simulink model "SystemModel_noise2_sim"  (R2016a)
settings: Solver=FixedStepAuto  StartTime=0.0  StopTime=Endtime  FixedStep=0.05  RelTol=1e-3
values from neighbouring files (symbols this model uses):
  alpha_AD = (2^n_AD - 1)/(V_AD_max - V_AD_min)    (= 204.6)    [SystemModel_noise2.m]    (also in SystemModel_noise1.m)
  alpha_PG = 100/(2^n_PG-1)    (= 0.392156862745)    [SystemModel_noise2.m]    (also in SystemModel_noise1.m)
  alpha_S_i = 5/37.5    (= 0.133333333333)    [SystemModel_noise2.m]    (also in MotorDriver_m.m; SystemModel_noise1.m)
  alpha_S_N = 1.5/1000    (= 0.0015)    [SystemModel_noise2.m]    (also in SystemModel_noise1.m)
  D_R = 6.0e-5    (= 6e-05)    [SystemModel_noise2.m]    (also in SystemModel_noise1.m)
  J_I = 1.3e-3    (= 0.0013)    [SystemModel_noise2.m]    (also in DCMotorDisk.m; SystemModel_noise1.m)
  J_M = 0.11e-3    (= 0.00011)    [SystemModel_noise2.m]    (also in DCMotorDisk.m; SystemModel_noise1.m)
  K_E = 7.16e-2    (= 0.0716)    [SystemModel_noise2.m]    (also in SystemModel_noise1.m)
  K_tau = 7.2e-2    (= 0.072)    [SystemModel_noise2.m]    (also in DCMotorDisk.m; SystemModel_noise1.m)
  kc = 0.1    [SystemModel_noise2.m]    (also in SystemModel_noise1.m = 0.05)
  L_E = 0.2    [SystemModel_noise2.m]    (also in SystemModel_noise1.m)
  n_PG = 8    [SystemModel_noise2.m]    (also in SystemModel_noise1.m)
  R_E = 5.7    [SystemModel_noise2.m]    (also in SystemModel_noise1.m)
  SV = 1000    [SystemModel_noise2.m]    (also in SystemModel_noise1.m)
  T_D = 0.1    [SystemModel_noise2.m]    (also in SystemModel_noise1.m = 0.01)
  T_I = 1.5    [SystemModel_noise2.m]    (also in SystemModel_noise1.m = 1.2)
  Tc = 1/(2*pi*fc)    (= 0.159154943092)    [SystemModel_noise2.m]
  u_max = 100    [SystemModel_noise2.m]    (also in Controller.m; SystemModel_noise1.m)
  u_min = 0    [SystemModel_noise2.m]    (also in Controller.m; SystemModel_noise1.m)
  V_AD_max = 5    [SystemModel_noise2.m]    (also in SystemModel_noise1.m)
  V_AD_min = 0    [SystemModel_noise2.m]    (also in SystemModel_noise1.m)
  Vs = 24    [SystemModel_noise2.m]    (also in MotorDriver.m; MotorDriver_m.m; SystemModel_noise1.m)

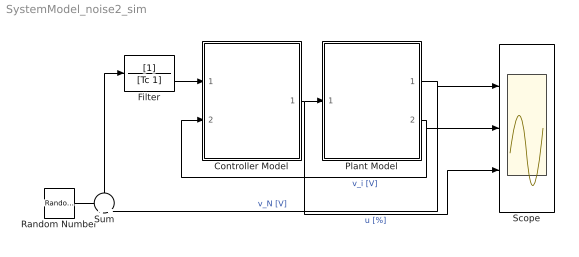
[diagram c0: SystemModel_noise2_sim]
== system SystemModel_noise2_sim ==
  Controller Model : Subsystem
  Filter : TransferFcn  Commented=through  Denominator=[Tc 1]
  Plant Model : Subsystem
  Random Number : RandomNumber  Variance=1e-2  SampleTime=0
  Scope : Scope  NumInputPorts=3
  Sum : Sum  Inputs=+|+
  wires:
  Controller Model/1(u_PG [%]) -> Scope/3, Plant Model/1(u_MD [%])  "u [%]"
  Plant Model/2(v_i [V]) -> Scope/2, Controller Model/2(v_i [V])  "v_i [V]"
  Plant Model/1(v_N [V]) -> Sum/2, Scope/1  "v_N [V]"
  Sum/1 -> Filter/1
  Random Number/1 -> Sum/1
  Filter/1 -> Controller Model/1(v_N [V])

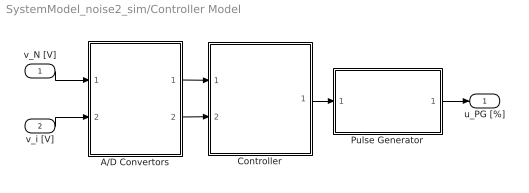
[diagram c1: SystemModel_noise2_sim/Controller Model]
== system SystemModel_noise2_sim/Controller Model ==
  v_N [V] : Inport
  v_i [V] : Inport  Port=2
  A/D Convertors : Subsystem
  Controller : Subsystem
  Pulse Generator : Subsystem
  u_PG [%] : Outport
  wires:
  v_i [V]/1 -> A/D Convertors/2(v_i [V])
  A/D Convertors/2(d_AD_i [-]) -> Controller/2(d_AD_i [-])
  Controller/1(d_PG [-]) -> Pulse Generator/1(d_PG [-])
  A/D Convertors/1(d_AD_N [-]) -> Controller/1(d_AD_N [-])
  Pulse Generator/1(u_PG [%]) -> u_PG [%]/1
  v_N [V]/1 -> A/D Convertors/1(v_N [V])

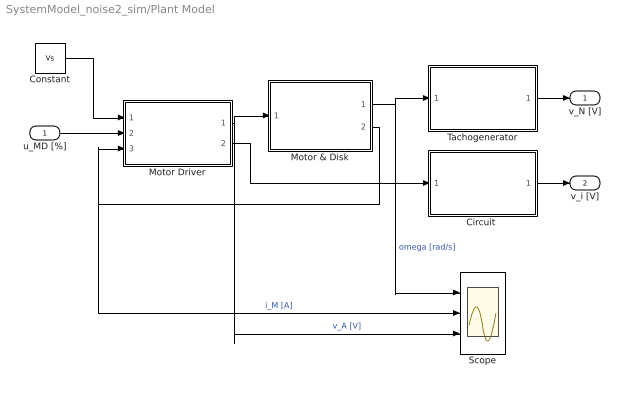
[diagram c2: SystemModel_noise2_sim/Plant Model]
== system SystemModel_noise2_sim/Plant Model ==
  u_MD [%] : Inport
  "Circuit " : Subsystem
  Constant : Constant  Value=Vs
  Motor & Disk : Subsystem
  Motor Driver : Subsystem
  Scope : Scope  NumInputPorts=3
  Tachogenerator : Subsystem
  v_N [V] : Outport
  v_i [V] : Outport  Port=2
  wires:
  Tachogenerator/1(v_N [V]) -> v_N [V]/1
  Motor Driver/1(v_A [V]) -> Scope/3, Motor & Disk/1(v_M [V])  "v_A [V]"
  Constant/1 -> Motor Driver/1(Vs [V])
  Motor & Disk/1(omega [rad/s]) -> Scope/1, Tachogenerator/1(omega [rad/s])  "omega [rad/s]"
  u_MD [%]/1 -> Motor Driver/2(u_MD [%])
  Motor & Disk/2(i_M [A]) -> Scope/2, Motor Driver/3(i_M [A])  "i_M [A]"
  Motor Driver/2(v_i [V]) -> "Circuit "/1(v_i [V])
  "Circuit "/1(v_i_st [V]) -> v_i [V]/1

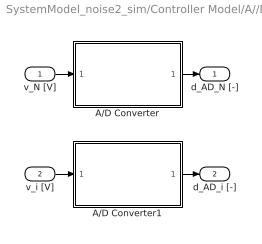
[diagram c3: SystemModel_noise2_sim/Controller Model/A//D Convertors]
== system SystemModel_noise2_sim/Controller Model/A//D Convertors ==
  v_N [V] : Inport
  v_i [V] : Inport  Port=2
  A/D Converter : Subsystem
  A/D Converter1 : Subsystem
  d_AD_N [-] : Outport
  d_AD_i [-] : Outport  Port=2
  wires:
  A/D Converter1/1(d_AD [-]) -> d_AD_i [-]/1
  v_N [V]/1 -> A/D Converter/1(v_AD [V])
  v_i [V]/1 -> A/D Converter1/1(v_AD [V])
  A/D Converter/1(d_AD [-]) -> d_AD_N [-]/1

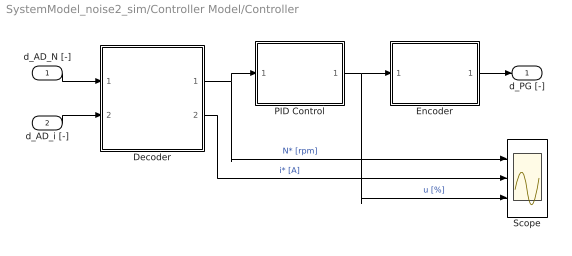
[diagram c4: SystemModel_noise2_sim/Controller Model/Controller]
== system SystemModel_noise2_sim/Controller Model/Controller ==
  d_AD_N [-] : Inport
  d_AD_i [-] : Inport  Port=2
  Decoder : Subsystem
  Encoder : Subsystem
  PID Control : Subsystem
  Scope : Scope  NumInputPorts=3
  d_PG [-] : Outport
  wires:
  d_AD_N [-]/1 -> Decoder/1(d_AD_N [-])
  Encoder/1(d_PG [-]) -> d_PG [-]/1
  Decoder/1(N* [rpm]) -> PID Control/1(N* [rpm]), Scope/1  "N* [rpm]"
  Decoder/2(i* [A]) -> Scope/2  "i* [A]"
  d_AD_i [-]/1 -> Decoder/2(d_AD_i [-])
  PID Control/1(u [%]) -> Scope/3, Encoder/1(u [%])  "u [%]"

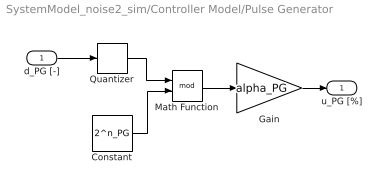
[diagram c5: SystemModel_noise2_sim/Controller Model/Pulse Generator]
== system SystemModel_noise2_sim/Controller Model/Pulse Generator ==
  d_PG [-] : Inport
  Constant : Constant  Value=2^n_PG
  Gain : Gain  Gain=alpha_PG
  Math Function : Math  Operator=mod
  Quantizer : Quantizer  QuantizationInterval=1
  u_PG [%] : Outport
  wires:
  d_PG [-]/1 -> Quantizer/1
  Quantizer/1 -> Math Function/1
  Gain/1 -> u_PG [%]/1
  Math Function/1 -> Gain/1
  Constant/1 -> Math Function/2

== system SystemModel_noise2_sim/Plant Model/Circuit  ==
  v_i [V] : Inport
  Saturation : Saturate  UpperLimit=5  LowerLimit=0
  v_i_st [V] : Outport
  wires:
  Saturation/1 -> v_i_st [V]/1
  v_i [V]/1 -> Saturation/1

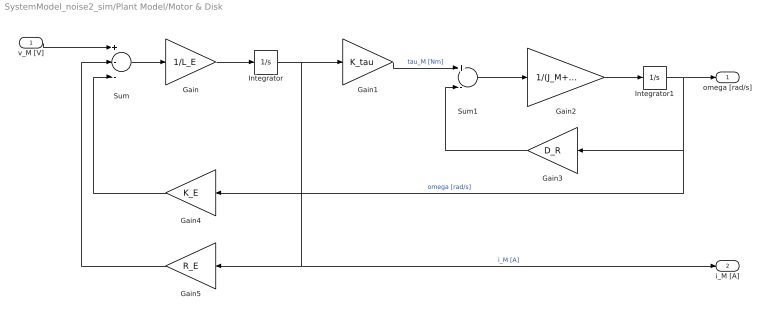
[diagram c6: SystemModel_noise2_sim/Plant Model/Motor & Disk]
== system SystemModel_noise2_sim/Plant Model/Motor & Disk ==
  v_M [V] : Inport
  Gain : Gain  Gain=1/L_E
  Gain1 : Gain  Gain=K_tau
  Gain2 : Gain  Gain=1/(J_M+J_I)
  Gain3 : Gain  Gain=D_R
  Gain4 : Gain  Gain=K_E
  Gain5 : Gain  Gain=R_E
  Integrator : Integrator
  Integrator1 : Integrator
  Sum : Sum  Inputs=+--
  Sum1 : Sum  Inputs=+-
  omega [rad/s] : Outport
  i_M [A] : Outport  Port=2
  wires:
  v_M [V]/1 -> Sum/1
  Sum/1 -> Gain/1
  Gain/1 -> Integrator/1
  Integrator/1 -> Gain1/1, i_M [A]/1, Gain5/1  "i_M [A]"
  Gain5/1 -> Sum/2
  Gain1/1 -> Sum1/1  "tau_M [Nm]"
  Sum1/1 -> Gain2/1
  Gain2/1 -> Integrator1/1
  Integrator1/1 -> Gain4/1, Gain3/1, omega [rad/s]/1  "omega [rad/s]"
  Gain4/1 -> Sum/3
  Gain3/1 -> Sum1/2

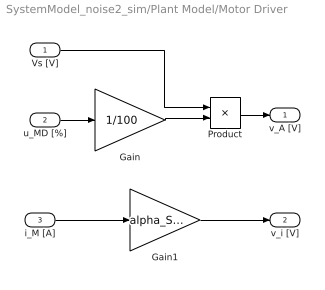
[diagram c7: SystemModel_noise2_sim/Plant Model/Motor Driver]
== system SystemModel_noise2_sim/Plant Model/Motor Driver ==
  Vs [V] : Inport
  u_MD [%] : Inport  Port=2
  i_M [A] : Inport  Port=3
  Gain : Gain  Gain=1/100
  Gain1 : Gain  Gain=alpha_S_i
  Product : Product
  v_A [V] : Outport
  v_i [V] : Outport  Port=2
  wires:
  u_MD [%]/1 -> Gain/1
  Product/1 -> v_A [V]/1
  Vs [V]/1 -> Product/1
  Gain/1 -> Product/2
  i_M [A]/1 -> Gain1/1
  Gain1/1 -> v_i [V]/1

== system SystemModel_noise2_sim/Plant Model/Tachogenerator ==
  omega [rad/s] : Inport
  Gain : Gain  Gain=60/(2*pi)
  Gain1 : Gain  Gain=alpha_S_N
  v_N [V] : Outport
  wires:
  omega [rad/s]/1 -> Gain/1
  Gain1/1 -> v_N [V]/1
  Gain/1 -> Gain1/1  "N [rpm]"

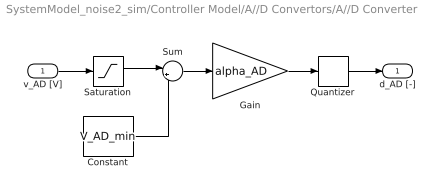
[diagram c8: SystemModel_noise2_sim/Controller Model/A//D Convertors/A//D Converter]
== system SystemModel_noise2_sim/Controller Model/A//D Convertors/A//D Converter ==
  v_AD [V] : Inport
  Constant : Constant  Value=V_AD_min
  Gain : Gain  Gain=alpha_AD
  Quantizer : Quantizer  QuantizationInterval=1
  Saturation : Saturate  UpperLimit=V_AD_max  LowerLimit=V_AD_min
  Sum : Sum  Inputs=|+-
  d_AD [-] : Outport
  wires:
  v_AD [V]/1 -> Saturation/1
  Gain/1 -> Quantizer/1
  Quantizer/1 -> d_AD [-]/1
  Sum/1 -> Gain/1
  Constant/1 -> Sum/2
  Saturation/1 -> Sum/1

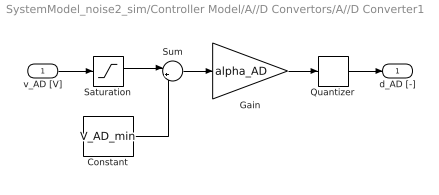
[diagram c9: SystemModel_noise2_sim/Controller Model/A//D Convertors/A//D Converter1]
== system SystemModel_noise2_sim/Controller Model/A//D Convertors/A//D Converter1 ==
  v_AD [V] : Inport
  Constant : Constant  Value=V_AD_min
  Gain : Gain  Gain=alpha_AD
  Quantizer : Quantizer  QuantizationInterval=1
  Saturation : Saturate  UpperLimit=V_AD_max  LowerLimit=V_AD_min
  Sum : Sum  Inputs=|+-
  d_AD [-] : Outport
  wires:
  v_AD [V]/1 -> Saturation/1
  Gain/1 -> Quantizer/1
  Quantizer/1 -> d_AD [-]/1
  Sum/1 -> Gain/1
  Constant/1 -> Sum/2
  Saturation/1 -> Sum/1

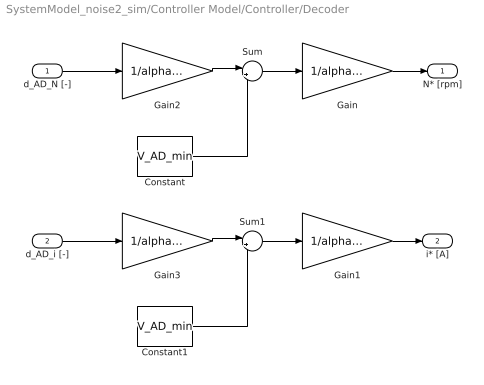
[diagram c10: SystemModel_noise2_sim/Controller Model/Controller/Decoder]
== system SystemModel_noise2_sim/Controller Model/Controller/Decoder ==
  d_AD_N [-] : Inport
  d_AD_i [-] : Inport  Port=2
  Constant : Constant  Value=V_AD_min
  Constant1 : Constant  Value=V_AD_min
  Gain : Gain  Gain=1/alpha_S_N
  Gain1 : Gain  Gain=1/alpha_S_i
  Gain2 : Gain  Gain=1/alpha_AD
  Gain3 : Gain  Gain=1/alpha_AD
  Sum : Sum  Inputs=|++
  Sum1 : Sum  Inputs=|++
  N* [rpm] : Outport
  i* [A] : Outport  Port=2
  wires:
  Gain/1 -> N* [rpm]/1
  d_AD_N [-]/1 -> Gain2/1
  Sum/1 -> Gain/1
  Constant/1 -> Sum/2
  Gain2/1 -> Sum/1
  Gain1/1 -> i* [A]/1
  d_AD_i [-]/1 -> Gain3/1
  Sum1/1 -> Gain1/1
  Constant1/1 -> Sum1/2
  Gain3/1 -> Sum1/1

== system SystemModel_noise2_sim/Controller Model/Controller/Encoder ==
  u [%] : Inport
  Constant1 : Constant  Value=u_min
  Gain1 : Gain  Gain=(2^n_PG-1)/(u_max-u_min)
  Sum : Sum  Inputs=|++
  d_PG [-] : Outport
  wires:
  u [%]/1 -> Sum/1
  Gain1/1 -> d_PG [-]/1
  Sum/1 -> Gain1/1
  Constant1/1 -> Sum/2

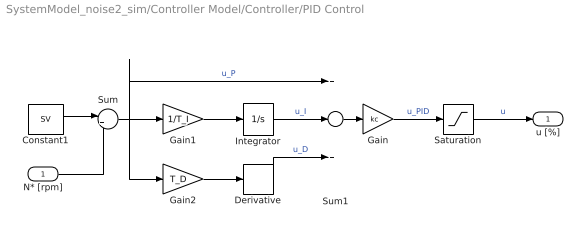
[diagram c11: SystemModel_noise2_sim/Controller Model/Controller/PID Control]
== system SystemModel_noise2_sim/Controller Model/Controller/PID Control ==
  N* [rpm] : Inport
  Constant1 : Constant  Value=SV
  Derivative : Derivative
  Gain : Gain  Gain=kc
  Gain1 : Gain  Gain=1/T_I
  Gain2 : Gain  Gain=T_D
  Integrator : Integrator
  Saturation : Saturate  UpperLimit=u_max  LowerLimit=u_min
  Sum : Sum  Inputs=|+-
  Sum1 : Sum  Inputs=+|+|+
  u [%] : Outport
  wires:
  Gain/1 -> Saturation/1  "u_PID"
  N* [rpm]/1 -> Sum/2
  Constant1/1 -> Sum/1
  Integrator/1 -> Sum1/2  "u_I"
  Gain1/1 -> Integrator/1
  Gain2/1 -> Derivative/1
  Sum1/1 -> Gain/1
  Saturation/1 -> u [%]/1  "u"
  Sum/1 -> Sum1/1, Gain2/1, Gain1/1  "u_P"
  Derivative/1 -> Sum1/3  "u_D"
